FUNCTION "FC_GRP_52" : VOID
TITLE =GROUP =52
{ S7_language := '9(1) Angielski (Stany Zjednoczone)  11.01.2022  09:45:15' }
VERSION : 0.1


VAR_TEMP
  CL : "UDT_CABINET";	//CABINET LOCAL
  CR : "UDT_CABINET";	//CABINET REMOTE
  RelError : BOOL ;	//ERROR RELEASE
  RelErrorCL : BOOL ;	//ERROR RELEASE FROM CABINET LOCAL
  RelErrorCR : BOOL ;	//ERROR RELEASE FROM CABINET REMOTE
  RelControl : BOOL ;	//CONTROL RELEASE
  RelControlCL : BOOL ;	//CONTROL RELEASE FROM CABINET LOCAL
  RelControlCR : BOOL ;	//CONTROL RELEASE FROM CABINET REMOTE
  ErrorConfirm : BOOL ;	//ERROR CONFIRM
  AutoOn : BOOL ;	//AUTOMATIC ON
  AutoOff : BOOL ;	//AUTOMATIC OFF
  RelAuto : BOOL ;	//AUTOMATIC RELEASE
  LAMP_ON : BOOL ;
  TempSetpoint : REAL ;
END_VAR
BEGIN
NETWORK
TITLE =GLOBAL SIGNALS
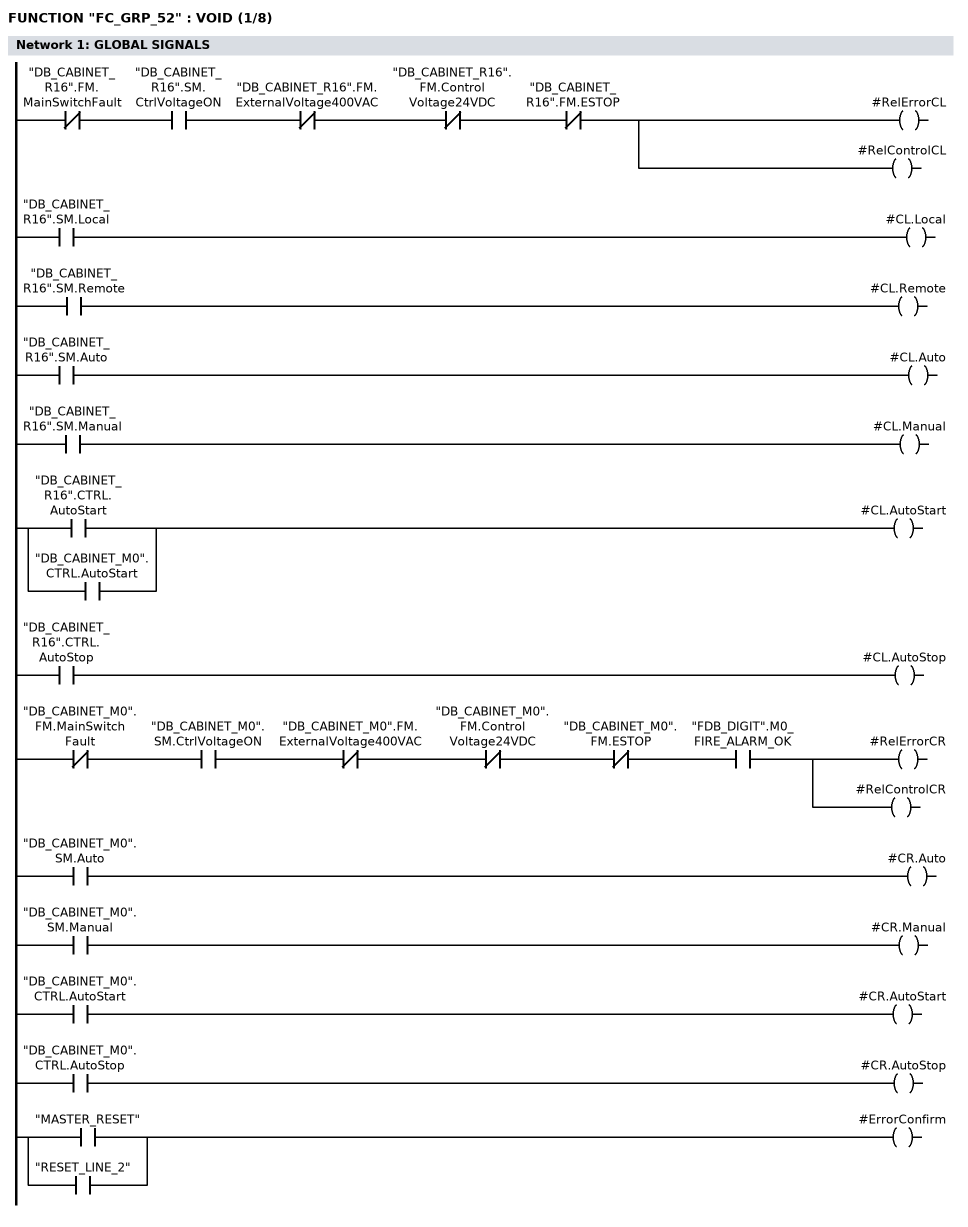
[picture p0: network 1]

//LOCAL
      UN    "DB_CABINET_R16".FM.MainSwitchFault;
      U     "DB_CABINET_R16".SM.CtrlVoltageON;
      UN    "DB_CABINET_R16".FM.ExternalVoltage400VAC;
      UN    "DB_CABINET_R16".FM.ControlVoltage24VDC;
      UN    "DB_CABINET_R16".FM.ESTOP;
      =     #RelErrorCL;
      =     #RelControlCL;

      U     "DB_CABINET_R16".SM.Local;
      =     #CL.Local;
      U     "DB_CABINET_R16".SM.Remote;
      =     #CL.Remote;
      U     "DB_CABINET_R16".SM.Auto;
      =     #CL.Auto;
      U     "DB_CABINET_R16".SM.Manual;
      =     #CL.Manual;
      U     "DB_CABINET_R16".CTRL.AutoStart;
      O     "DB_CABINET_M0".CTRL.AutoStart;
      =     #CL.AutoStart;
      U     "DB_CABINET_R16".CTRL.AutoStop;
      =     #CL.AutoStop;


//REMOTE

      UN    "DB_CABINET_M0".FM.MainSwitchFault;
      U     "DB_CABINET_M0".SM.CtrlVoltageON;
      UN    "DB_CABINET_M0".FM.ExternalVoltage400VAC;
      UN    "DB_CABINET_M0".FM.ControlVoltage24VDC;
//      UN    "DB_CABINET_M0".FM.ControlVoltage230VAC_MS
      UN    "DB_CABINET_M0".FM.ESTOP;
      U     "FDB_DIGIT".M0_FIRE_ALARM_OK;
      =     #RelErrorCR;
      =     #RelControlCR;

      U     "DB_CABINET_M0".SM.Auto;
      =     #CR.Auto;
      U     "DB_CABINET_M0".SM.Manual;
      =     #CR.Manual;
      U     "DB_CABINET_M0".CTRL.AutoStart;
      =     #CR.AutoStart;
      U     "DB_CABINET_M0".CTRL.AutoStop;
      =     #CR.AutoStop;


      U     "MASTER_RESET";
      O     "RESET_LINE_2";
      =     #ErrorConfirm;

NETWORK
TITLE =GLOBAL SIGNALS - GROUP GENERAL ERROR AND WARNING
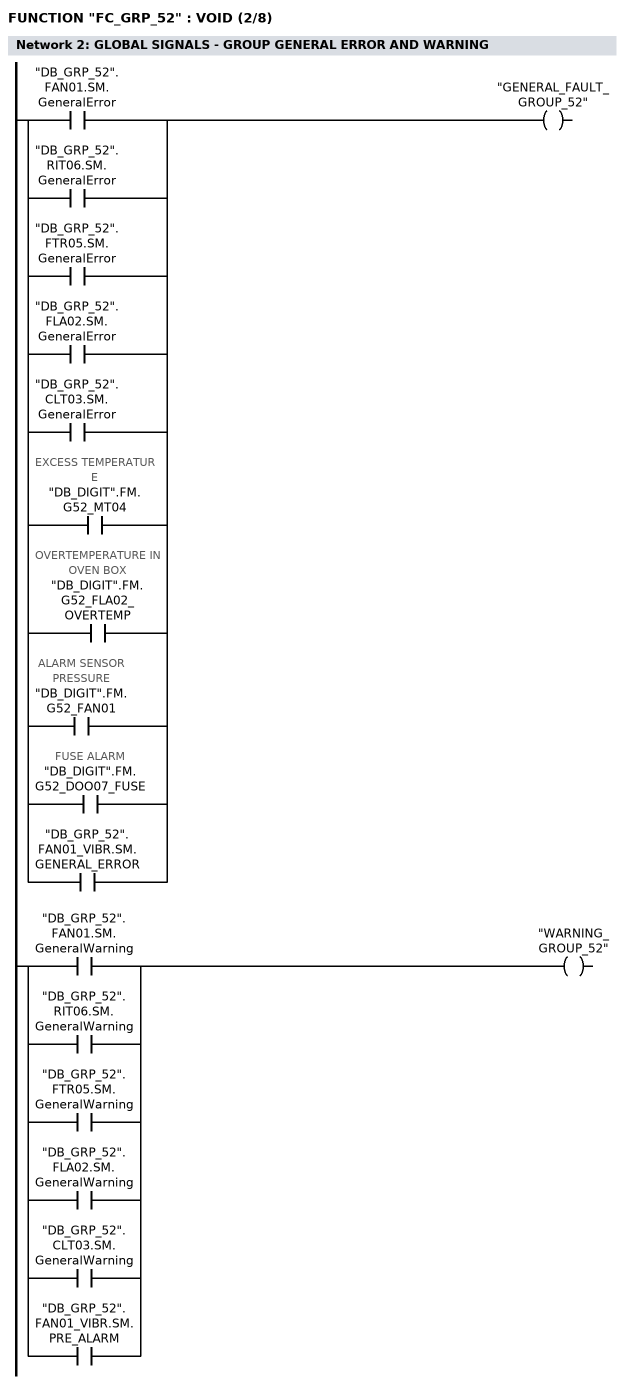
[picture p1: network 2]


      U     "DB_GRP_52".FAN01.SM.GeneralError;
      O     "DB_GRP_52".RIT06.SM.GeneralError;
      O     "DB_GRP_52".FTR05.SM.GeneralError;
      O     "DB_GRP_52".FLA02.SM.GeneralError;
      O     "DB_GRP_52".CLT03.SM.GeneralError;
      O     "DB_DIGIT".FM.G52_MT04; //EXCESS TEMPERATURE
      O     "DB_DIGIT".FM.G52_FLA02_OVERTEMP; //OVERTEMPERATURE IN OVEN BOX
      O     "DB_DIGIT".FM.G52_FAN01; //ALARM SENSOR PRESSURE
      O     "DB_DIGIT".FM.G52_DOO07_FUSE; //FUSE ALARM
      O     "DB_GRP_52".FAN01_VIBR.SM.GENERAL_ERROR;
      =     "GENERAL_FAULT_GROUP_52";

      U     "DB_GRP_52".FAN01.SM.GeneralWarning;
      O     "DB_GRP_52".RIT06.SM.GeneralWarning;
      O     "DB_GRP_52".FTR05.SM.GeneralWarning;
      O     "DB_GRP_52".FLA02.SM.GeneralWarning;
      O     "DB_GRP_52".CLT03.SM.GeneralWarning;
      O     "DB_GRP_52".FAN01_VIBR.SM.PRE_ALARM;
      =     "WARNING_GROUP_52";


NETWORK
TITLE =RELEASE CONTROL
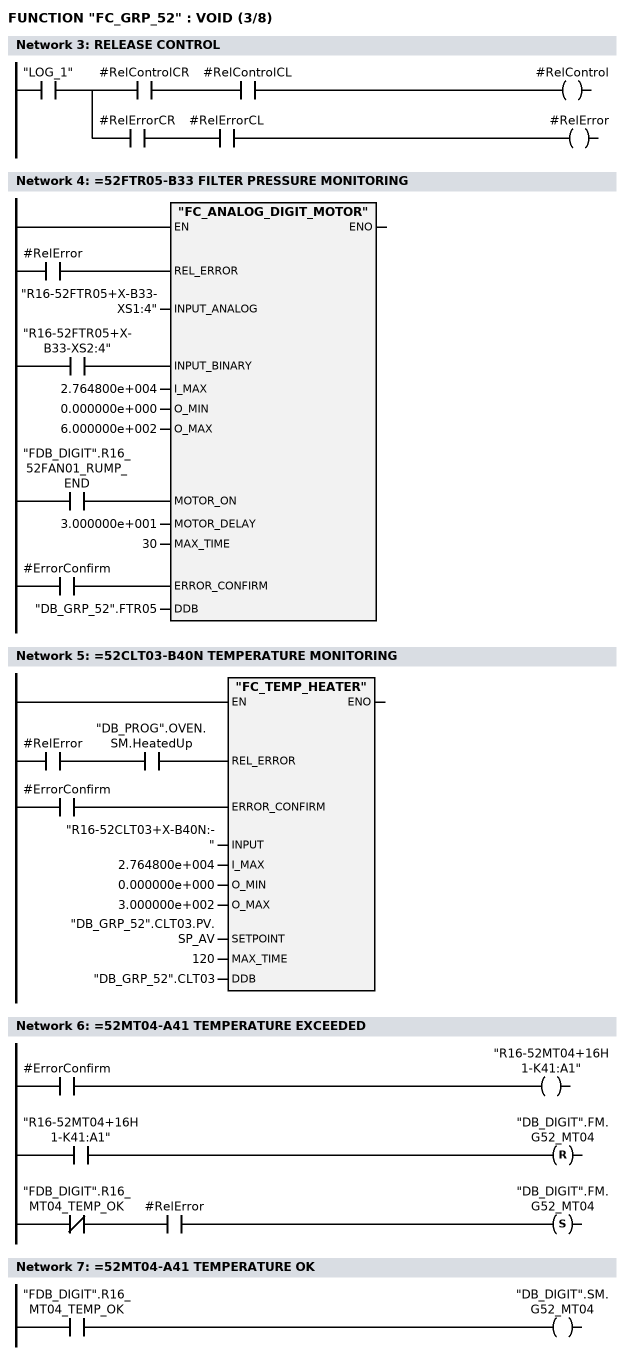
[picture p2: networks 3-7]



      U     "LOG_1";
      =     L     10.0;
      U     L     10.0;
      U     #RelControlCR;
      U     #RelControlCL;
      =     #RelControl;
      U     L     10.0;
      U     #RelErrorCR;
      U     #RelErrorCL;
      =     #RelError;
NETWORK
TITLE ==52FTR05-B33 FILTER PRESSURE MONITORING

      U     #RelError;
      =     L     10.0;
      BLD   103;
      U     "R16-52FTR05+X-B33-XS2:4";
      =     L     10.1;
      BLD   103;
      U     "FDB_DIGIT".R16_52FAN01_RUMP_END;
      =     L     10.2;
      BLD   103;
      U     #ErrorConfirm;
      =     L     10.3;
      BLD   103;
      CALL "FC_ANALOG_DIGIT_MOTOR" (
           REL_ERROR                := L     10.0,
           INPUT_ANALOG             := "R16-52FTR05+X-B33-XS1:4",
           INPUT_BINARY             := L     10.1,
           I_MAX                    := 2.764800e+004,
           O_MIN                    := 0.000000e+000,
           O_MAX                    := 6.000000e+002,
           MOTOR_ON                 := L     10.2,
           MOTOR_DELAY              := 3.000000e+001,
           MAX_TIME                 := 30,
           ERROR_CONFIRM            := L     10.3,
           DDB                      := "DB_GRP_52".FTR05);
      NOP   0;
NETWORK
TITLE ==52CLT03-B40N TEMPERATURE MONITORING

      U     #RelError;
      U     "DB_PROG".OVEN.SM.HeatedUp;
      =     L     10.0;
      BLD   103;
      U     #ErrorConfirm;
      =     L     10.1;
      BLD   103;
      CALL "FC_TEMP_HEATER" (
           REL_ERROR                := L     10.0,
           ERROR_CONFIRM            := L     10.1,
           INPUT                    := "R16-52CLT03+X-B40N:-",
           I_MAX                    := 2.764800e+004,
           O_MIN                    := 0.000000e+000,
           O_MAX                    := 3.000000e+002,
           SETPOINT                 := "DB_GRP_52".CLT03.PV.SP_AV,
           MAX_TIME                 := 120,
           DDB                      := "DB_GRP_52".CLT03);
      NOP   0;
NETWORK
TITLE ==52MT04-A41 TEMPERATURE EXCEEDED

      U     #ErrorConfirm;
      =     "R16-52MT04+16H1-K41:A1";
      U     "R16-52MT04+16H1-K41:A1";
      R     "DB_DIGIT".FM.G52_MT04;
      UN    "FDB_DIGIT".R16_MT04_TEMP_OK;
      U     #RelError;
      S     "DB_DIGIT".FM.G52_MT04;
      NOP   0;
NETWORK
TITLE ==52MT04-A41 TEMPERATURE OK

      U     "FDB_DIGIT".R16_MT04_TEMP_OK;
      =     "DB_DIGIT".SM.G52_MT04;
NETWORK
TITLE ==52DOO07-F1.1 ACCESS DOOR FUSE ERROR
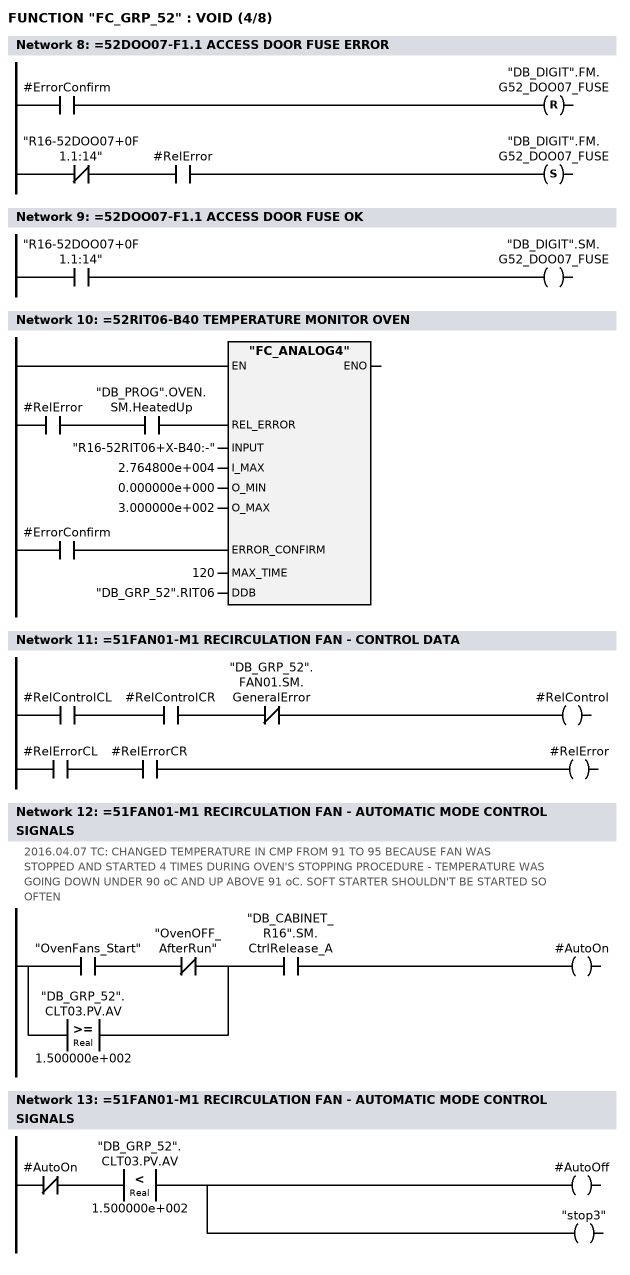
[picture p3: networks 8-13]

      U     #ErrorConfirm;
      R     "DB_DIGIT".FM.G52_DOO07_FUSE;
      UN    "R16-52DOO07+0F1.1:14";
      U     #RelError;
      S     "DB_DIGIT".FM.G52_DOO07_FUSE;
      NOP   0;
NETWORK
TITLE ==52DOO07-F1.1 ACCESS DOOR FUSE OK

      U     "R16-52DOO07+0F1.1:14";
      =     "DB_DIGIT".SM.G52_DOO07_FUSE;
NETWORK
TITLE ==52RIT06-B40 TEMPERATURE MONITOR OVEN

      U     #RelError;
      U     "DB_PROG".OVEN.SM.HeatedUp;
      =     L     10.0;
      BLD   103;
      U     #ErrorConfirm;
      =     L     10.1;
      BLD   103;
      CALL "FC_ANALOG4" (
           REL_ERROR                := L     10.0,
           INPUT                    := "R16-52RIT06+X-B40:-",
           I_MAX                    := 2.764800e+004,
           O_MIN                    := 0.000000e+000,
           O_MAX                    := 3.000000e+002,
           ERROR_CONFIRM            := L     10.1,
           MAX_TIME                 := 120,
           DDB                      := "DB_GRP_52".RIT06);
      NOP   0;
NETWORK
TITLE ==51FAN01-M1 RECIRCULATION FAN - CONTROL DATA

      U     #RelControlCL;
      U     #RelControlCR;
      UN    "DB_GRP_52".FAN01.SM.GeneralError;
      =     #RelControl;


      U     #RelErrorCL;
      U     #RelErrorCR;
      =     #RelError;
NETWORK
TITLE ==51FAN01-M1 RECIRCULATION FAN - AUTOMATIC MODE CONTROL SIGNALS
//2016.04.07 TC: CHANGED TEMPERATURE IN CMP FROM 91 TO 95 BECAUSE FAN WAS
//STOPPED AND STARTED 4 TIMES DURING OVEN'S STOPPING PROCEDURE - TEMPERATURE WAS
//GOING DOWN UNDER 90 oC AND UP ABOVE 91 oC. SOFT STARTER SHOULDN'T BE STARTED SO
//OFTEN
      U(    ;
      U     "OvenFans_Start";
      UN    "OvenOFF_AfterRun";
      O(    ;
      L     "DB_GRP_52".CLT03.PV.AV;
      L     1.500000e+002;
      >=R   ;
      )     ;
      )     ;
      U     "DB_CABINET_R16".SM.CtrlRelease_A;
      =     #AutoOn;
NETWORK
TITLE ==51FAN01-M1 RECIRCULATION FAN - AUTOMATIC MODE CONTROL SIGNALS

      UN    #AutoOn;
      U(    ;
      L     "DB_GRP_52".CLT03.PV.AV;
      L     1.500000e+002;
      <R    ;
      )     ;
      =     #AutoOff;
      =     "stop3";
NETWORK
TITLE ==52FAN01-A1 RECIRCULATION FAN
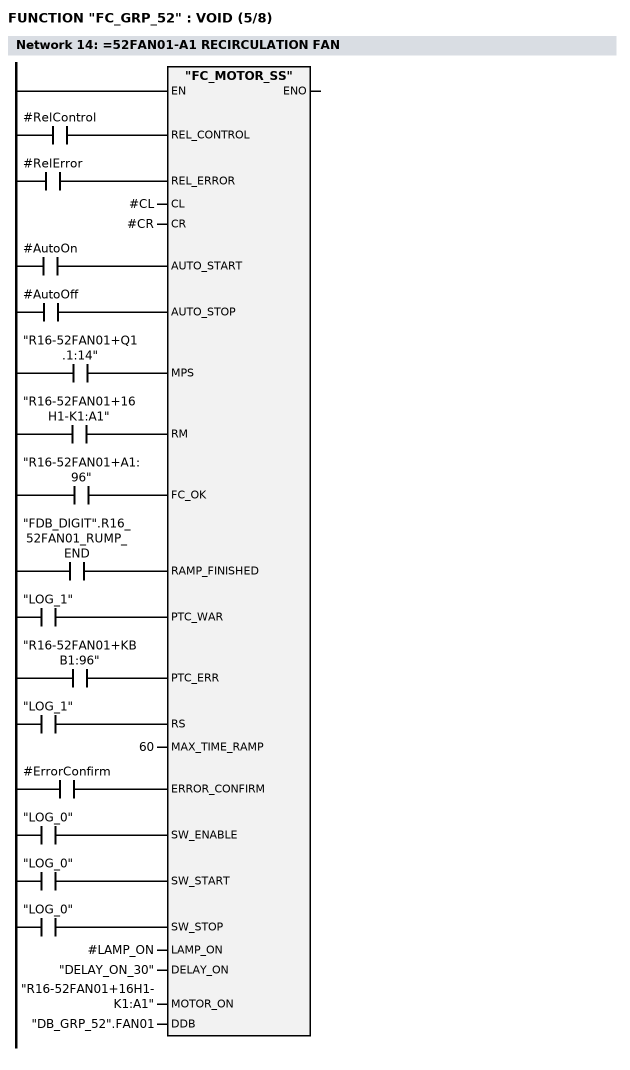
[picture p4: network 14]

      U     #RelControl;
      =     L     10.0;
      BLD   103;
      U     #RelError;
      =     L     10.1;
      BLD   103;
      U     #AutoOn;
      =     L     10.2;
      BLD   103;
      U     #AutoOff;
      =     L     10.3;
      BLD   103;
      U     "R16-52FAN01+Q1.1:14";
      =     L     10.4;
      BLD   103;
      U     "R16-52FAN01+16H1-K1:A1";
      =     L     10.5;
      BLD   103;
      U     "R16-52FAN01+A1:96";
      =     L     10.6;
      BLD   103;
      U     "FDB_DIGIT".R16_52FAN01_RUMP_END;
      =     L     10.7;
      BLD   103;
      U     "LOG_1";
      =     L     11.0;
      BLD   103;
      U     "R16-52FAN01+KBB1:96";
      =     L     11.1;
      BLD   103;
      U     "LOG_1";
      =     L     11.2;
      BLD   103;
      U     #ErrorConfirm;
      =     L     11.3;
      BLD   103;
      U     "LOG_0";
      =     L     11.4;
      BLD   103;
      U     "LOG_0";
      =     L     11.5;
      BLD   103;
      U     "LOG_0";
      =     L     11.6;
      BLD   103;
      CALL "FC_MOTOR_SS" (
           REL_CONTROL              := L     10.0,
           REL_ERROR                := L     10.1,
           CL                       := #CL,
           CR                       := #CR,
           AUTO_START               := L     10.2,
           AUTO_STOP                := L     10.3,
           MPS                      := L     10.4,
           RM                       := L     10.5,
           FC_OK                    := L     10.6,
           RAMP_FINISHED            := L     10.7,
           PTC_WAR                  := L     11.0,
           PTC_ERR                  := L     11.1,
           RS                       := L     11.2,
           MAX_TIME_RAMP            := 60,
           ERROR_CONFIRM            := L     11.3,
           SW_ENABLE                := L     11.4,
           SW_START                 := L     11.5,
           SW_STOP                  := L     11.6,
           LAMP_ON                  := #LAMP_ON,
           DELAY_ON                 := "DELAY_ON_30",
           MOTOR_ON                 := "R16-52FAN01+16H1-K1:A1",
           DDB                      := "DB_GRP_52".FAN01);
      NOP   0;
NETWORK
TITLE ==52FAN01 - S32F RECIRCULATION FAN PRESSURE OK
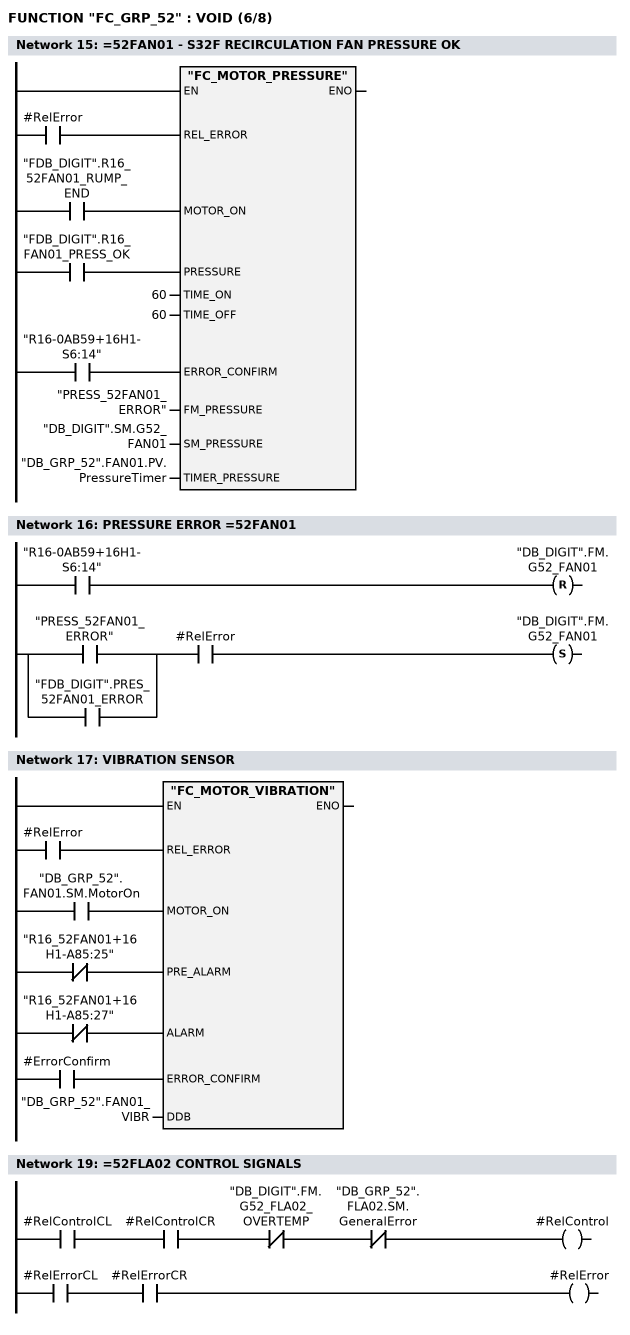
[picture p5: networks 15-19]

      U     #RelError;
      =     L     10.0;
      BLD   103;
      U     "FDB_DIGIT".R16_52FAN01_RUMP_END;
      =     L     10.1;
      BLD   103;
      U     "FDB_DIGIT".R16_FAN01_PRESS_OK;
      =     L     10.2;
      BLD   103;
      U     "R16-0AB59+16H1-S6:14";
      =     L     10.3;
      BLD   103;
      CALL "FC_MOTOR_PRESSURE" (
           REL_ERROR                := L     10.0,
           MOTOR_ON                 := L     10.1,
           PRESSURE                 := L     10.2,
           TIME_ON                  := 60,
           TIME_OFF                 := 60,
           ERROR_CONFIRM            := L     10.3,
           FM_PRESSURE              := "PRESS_52FAN01_ERROR",
           SM_PRESSURE              := "DB_DIGIT".SM.G52_FAN01,
           TIMER_PRESSURE           := "DB_GRP_52".FAN01.PV.PressureTimer);
      NOP   0;
NETWORK
TITLE =PRESSURE ERROR =52FAN01

      U     "R16-0AB59+16H1-S6:14";
      R     "DB_DIGIT".FM.G52_FAN01;
      U(    ;
      O     "PRESS_52FAN01_ERROR";
      O     "FDB_DIGIT".PRES_52FAN01_ERROR;
      )     ;
      U     #RelError;
      S     "DB_DIGIT".FM.G52_FAN01;
      NOP   0;
NETWORK
TITLE =VIBRATION SENSOR

      U     #RelError;
      =     L     10.0;
      BLD   103;
      U     "DB_GRP_52".FAN01.SM.MotorOn;
      =     L     10.1;
      BLD   103;
      UN    "R16_52FAN01+16H1-A85:25";
      =     L     10.2;
      BLD   103;
      UN    "R16_52FAN01+16H1-A85:27";
      =     L     10.3;
      BLD   103;
      U     #ErrorConfirm;
      =     L     10.4;
      BLD   103;
      CALL "FC_MOTOR_VIBRATION" (
           REL_ERROR                := L     10.0,
           MOTOR_ON                 := L     10.1,
           PRE_ALARM                := L     10.2,
           ALARM                    := L     10.3,
           ERROR_CONFIRM            := L     10.4,
           DDB                      := "DB_GRP_52".FAN01_VIBR);
      NOP   0;
NETWORK
TITLE =*********** 52FLA02 ******************

NETWORK
TITLE ==52FLA02 CONTROL SIGNALS

      U     #RelControlCL;
      U     #RelControlCR;
      UN    "DB_DIGIT".FM.G52_FLA02_OVERTEMP;
      UN    "DB_GRP_52".FLA02.SM.GeneralError;
      =     #RelControl;


      U     #RelErrorCL;
      U     #RelErrorCR;
      =     #RelError;


NETWORK
TITLE ==52FLA02, CONTROL SIGNALS - AUTO_ON
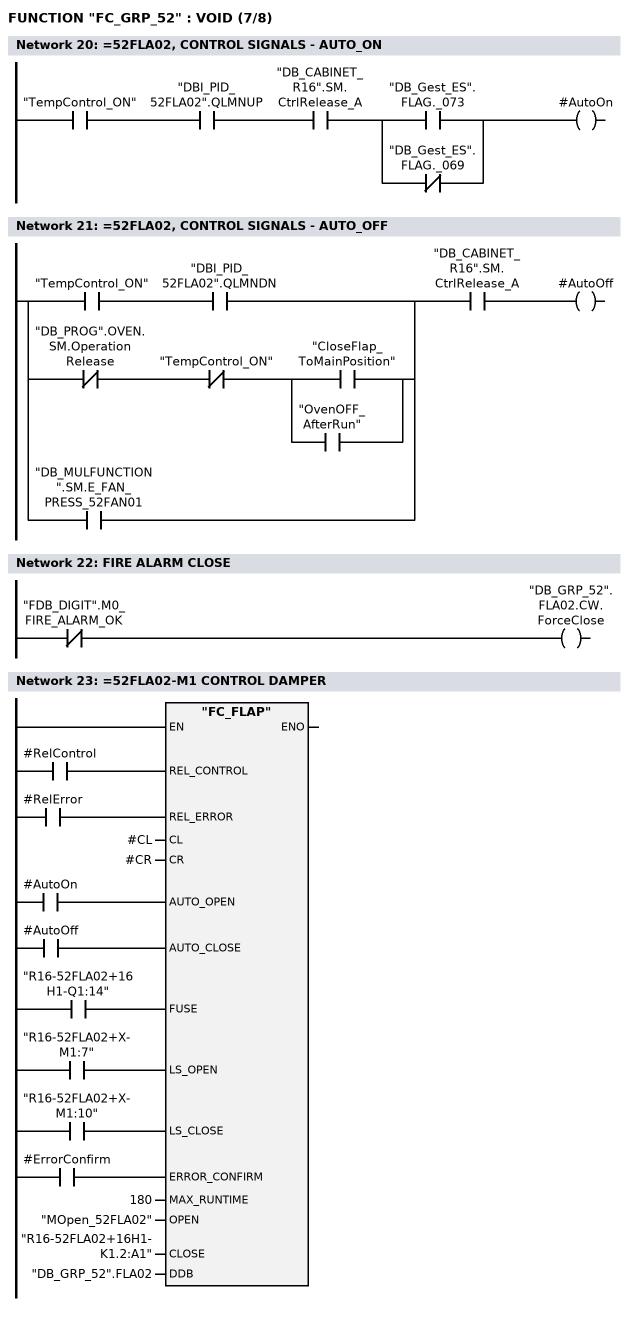
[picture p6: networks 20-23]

      U     "TempControl_ON";
      U     "DBI_PID_52FLA02".QLMNUP;
      U     "DB_CABINET_R16".SM.CtrlRelease_A;
      U(    ;
      O     "DB_Gest_ES".FLAG._073;
      ON    "DB_Gest_ES".FLAG._069;
      )     ;
      =     #AutoOn;
NETWORK
TITLE ==52FLA02, CONTROL SIGNALS - AUTO_OFF

      U(    ;
      U     "TempControl_ON";
      U     "DBI_PID_52FLA02".QLMNDN;
      O     ;
      UN    "DB_PROG".OVEN.SM.OperationRelease;
      UN    "TempControl_ON";
      U(    ;
      O     "CloseFlap_ToMainPosition";
      O     "OvenOFF_AfterRun";
      )     ;
      O     "DB_MULFUNCTION".SM.E_FAN_PRESS_52FAN01;
      )     ;
      U     "DB_CABINET_R16".SM.CtrlRelease_A;
      =     #AutoOff;
NETWORK
TITLE =FIRE ALARM CLOSE

      UN    "FDB_DIGIT".M0_FIRE_ALARM_OK;
      =     "DB_GRP_52".FLA02.CW.ForceClose;
NETWORK
TITLE ==52FLA02-M1 CONTROL DAMPER



      U     #RelControl;
      =     L     10.0;
      BLD   103;
      U     #RelError;
      =     L     10.1;
      BLD   103;
      U     #AutoOn;
      =     L     10.2;
      BLD   103;
      U     #AutoOff;
      =     L     10.3;
      BLD   103;
      U     "R16-52FLA02+16H1-Q1:14";
      =     L     10.4;
      BLD   103;
      U     "R16-52FLA02+X-M1:7";
      =     L     10.5;
      BLD   103;
      U     "R16-52FLA02+X-M1:10";
      =     L     10.6;
      BLD   103;
      U     #ErrorConfirm;
      =     L     10.7;
      BLD   103;
      CALL "FC_FLAP" (
           REL_CONTROL              := L     10.0,
           REL_ERROR                := L     10.1,
           CL                       := #CL,
           CR                       := #CR,
           AUTO_OPEN                := L     10.2,
           AUTO_CLOSE               := L     10.3,
           FUSE                     := L     10.4,
           LS_OPEN                  := L     10.5,
           LS_CLOSE                 := L     10.6,
           ERROR_CONFIRM            := L     10.7,
           MAX_RUNTIME              := 180,
           OPEN                     := "MOpen_52FLA02",
           CLOSE                    := "R16-52FLA02+16H1-K1.2:A1",
           DDB                      := "DB_GRP_52".FLA02);
      NOP   0;
NETWORK
TITLE =MANUAL INTERLOCKS - OPEN 43FLA02
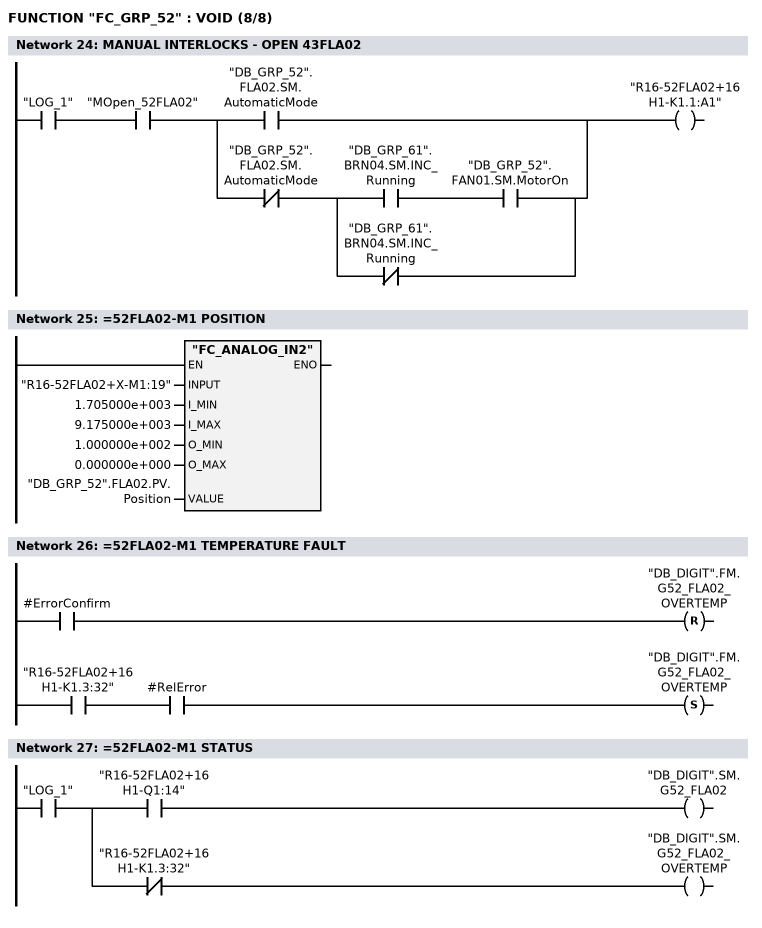
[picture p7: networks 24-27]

      U     "LOG_1";
      U     "MOpen_52FLA02";
      U(    ;
      O     "DB_GRP_52".FLA02.SM.AutomaticMode;
      O     ;
      UN    "DB_GRP_52".FLA02.SM.AutomaticMode;
      U(    ;
      U     "DB_GRP_61".BRN04.SM.INC_Running;
      U     "DB_GRP_52".FAN01.SM.MotorOn;
      ON    "DB_GRP_61".BRN04.SM.INC_Running;
      )     ;
      )     ;
      =     "R16-52FLA02+16H1-K1.1:A1";
NETWORK
TITLE ==52FLA02-M1 POSITION

      CALL "FC_ANALOG_IN2" (
           INPUT                    := "R16-52FLA02+X-M1:19",
           I_MIN                    := 1.705000e+003,
           I_MAX                    := 9.175000e+003,
           O_MIN                    := 1.000000e+002,
           O_MAX                    := 0.000000e+000,
           VALUE                    := "DB_GRP_52".FLA02.PV.Position);
      NOP   0;
NETWORK
TITLE ==52FLA02-M1 TEMPERATURE FAULT

      U     #ErrorConfirm;
      R     "DB_DIGIT".FM.G52_FLA02_OVERTEMP;
      U     "R16-52FLA02+16H1-K1.3:32";
      U     #RelError;
      S     "DB_DIGIT".FM.G52_FLA02_OVERTEMP;
      NOP   0;
NETWORK
TITLE ==52FLA02-M1 STATUS

      U     "LOG_1";
      =     L     10.0;
      U     L     10.0;
      U     "R16-52FLA02+16H1-Q1:14";
      =     "DB_DIGIT".SM.G52_FLA02;
      U     L     10.0;
      UN    "R16-52FLA02+16H1-K1.3:32";
      =     "DB_DIGIT".SM.G52_FLA02_OVERTEMP;
NETWORK
TITLE =END

END_FUNCTION

